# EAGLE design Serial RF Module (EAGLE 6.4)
DESCRIPTION: microOBD 200 OBD-II Module; HW_REV: 1.4; PCB_REV: C; PCB_SPEC1: Layer Count: 4; PCB_SPEC2: Size: 1.3" x 0.59"; PCB_SPEC3: Finish Thickness: 0.049" - 0.052"; PCB_SPEC4: Copper Weight: 1oz; TITLE: STM1120

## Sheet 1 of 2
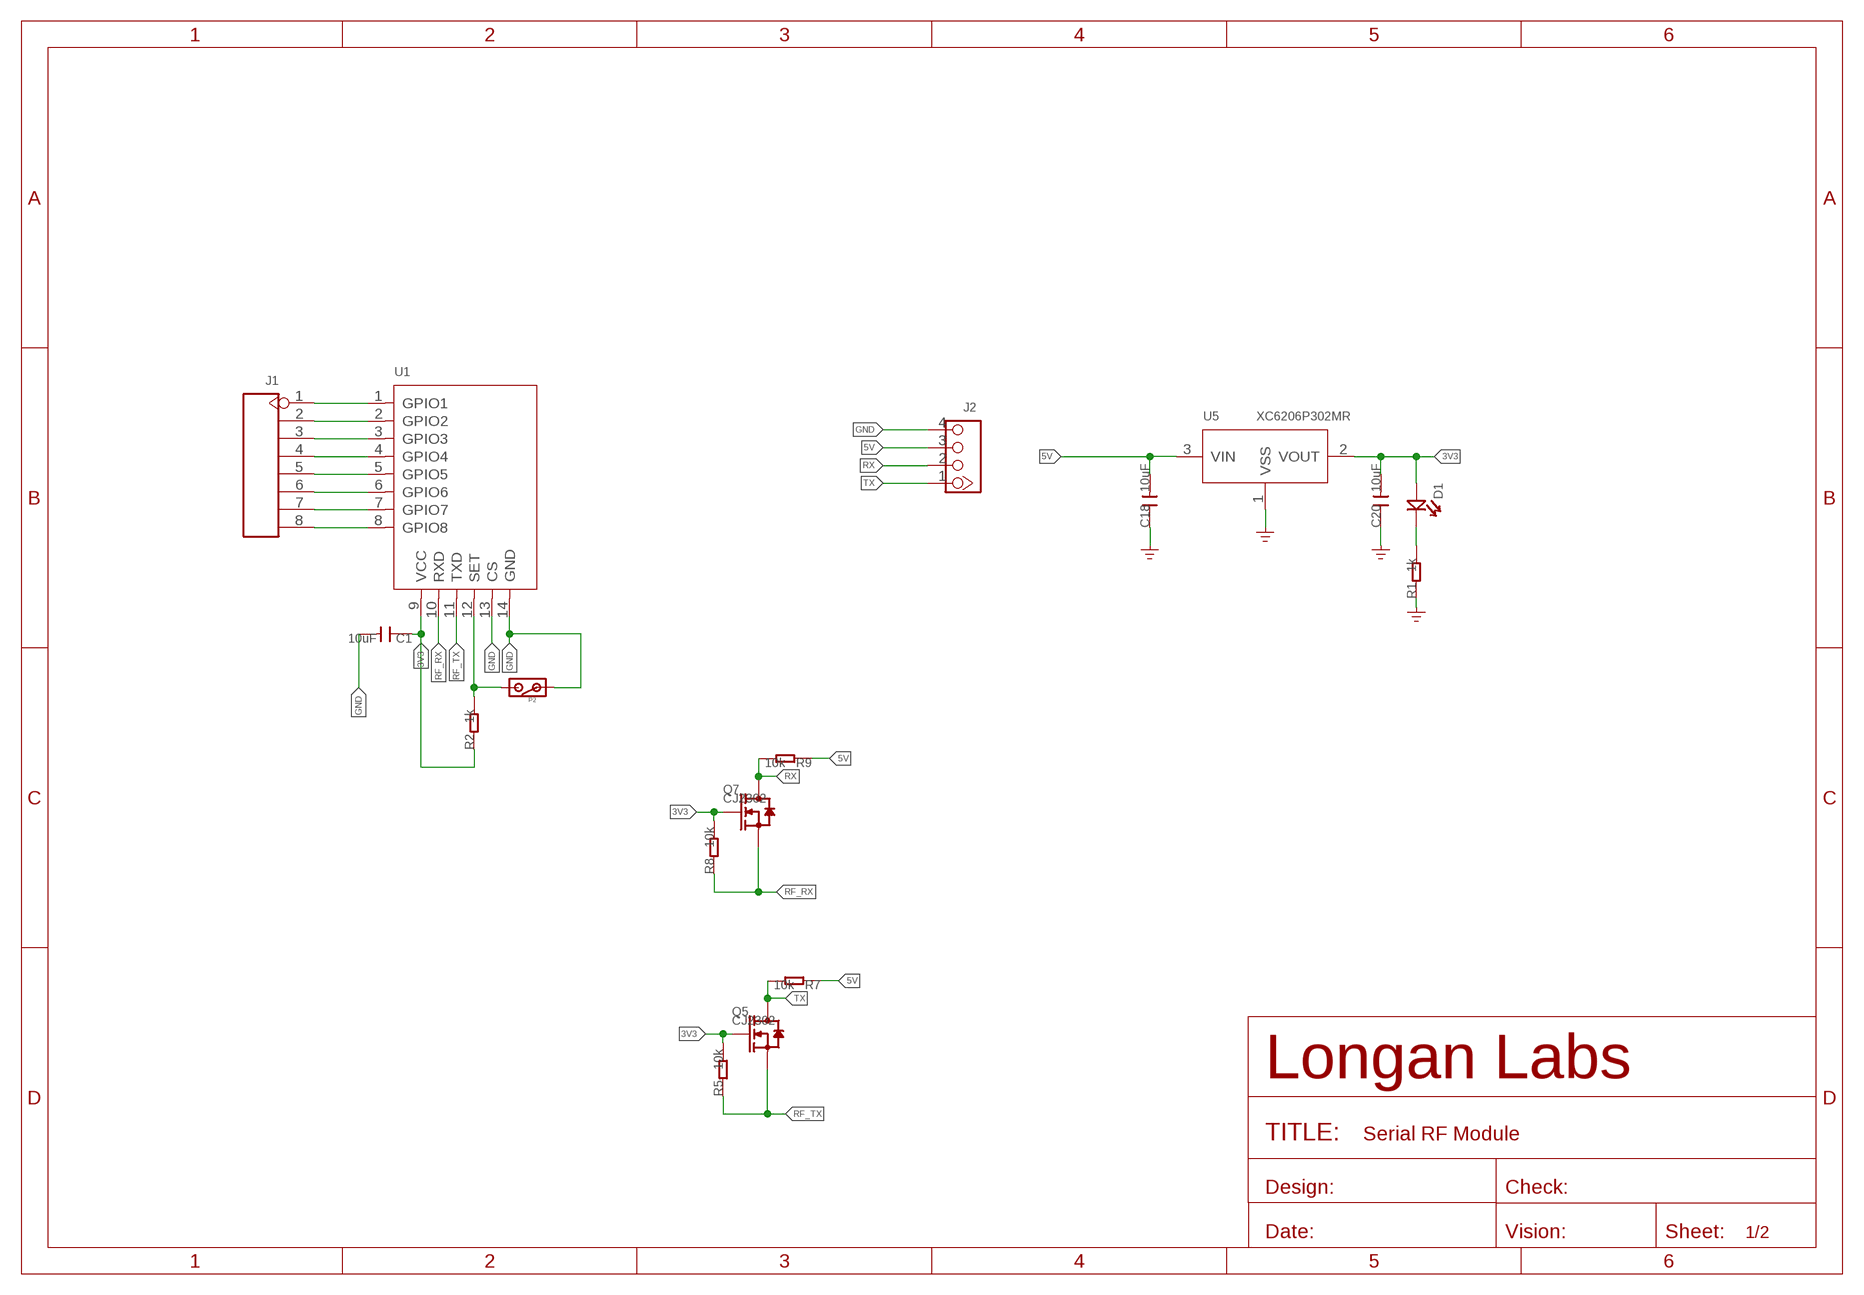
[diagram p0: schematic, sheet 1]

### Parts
C1  10uF  CAP-0603  [C0603]
C18  10uF  CAP-0603  [C0603]
C20  10uF  CAP-0603  [C0603]
D1  LED'0603'  [LED-0603]
J1  HEADER-8P-2.0-TEST  [H8-SMD-2.0-TEST]
J2  320110033  GROVE-CONNECTOR-DIP-2.0  [HW4-2.0]
P2  PAD-JUMPER-2P  [2P-SMD-1.78X1.27]
Q5  CJ2302  MOSFET-N'SOT23'  [SOT23]
Q7  CJ2302  MOSFET-N'SOT23'  [SOT23]
R1  1k  R-0603  [R0603]
R2  1k  R-0603  [R0603]
R5  10k  R-0603  [R0603]
R7  10k  R-0603  [R0603]
R8  10k  R-0603  [R0603]
R9  10k  R-0603  [R0603]
U1  MOUDLE-WIRELESS-SERIAL-JDY-40  [MOUDLE14P-1.5-23X13.7MM]
U5  XC6206P302MR  PMIC-XC6206PMR  [SOT-23]

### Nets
3V3: C1.1 C20.2 D1.+ Q5.1(G) Q7.1(G) R2.1 R5.2 R8.2 U1.9(VCC) U5.2(VOUT)
5V: C18.2 J2.3 R7.1 R9.1 U5.3(VIN)
GND: C1.2 C18.1 C20.1 J2.4 P2.1 R1.1 U1.13(CS) U1.14(GND) U5.1(VSS) ; supply symbol labelled GND_POWER
N$1: D1.- R1.2
N$2: P2.2 R2.2 U1.12(SET)
N$3: J1.1 U1.1(GPIO1)
N$4: J1.2 U1.2(GPIO2)
N$5: J1.3 U1.3(GPIO3)
N$6: J1.4 U1.4(GPIO4)
N$7: J1.5 U1.5(GPIO5)
N$8: J1.6 U1.6(GPIO6)
N$9: J1.7 U1.7(GPIO7)
N$10: J1.8 U1.8(GPIO8)
RF_RX: Q7.2(S) R8.1 U1.10(RXD)
RF_TX: Q5.2(S) R5.1 U1.11(TXD)
RX: J2.2 Q7.3(D) R9.2
TX: J2.1 Q5.3(D) R7.2

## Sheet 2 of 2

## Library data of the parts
C1 C18 C20 = Discrete-new:CAP: Ceramic Capacitors
D1 = Discrete-new:LED
J1 = Connector-new:HEADER-8P
J2 = Connector-new:GROVE-CONNECTOR-DIP: 4P-2.0:320110033;4P-2.0-90D:320110034
P2 = Discrete:PAD-JUMPER-2P
Q5 Q7 = Discrete:MOSFET-N: IRLL014: http://www.vishay.com/docs/91319/sihll014.pdf
R1 R2 R5 R7-R9 = Discrete:R*
U1 = Longan-moudle:MOUDLE-WIRELESS-SERIAL-JDY-40
U5 = IC-new:PMIC-XC6206P: LOW ESR Cap.Compatible Positive Voltage Regulators

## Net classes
3 usbvcc: width 0.152 mm, drill 0.152 mm, clearance 0.152 mm

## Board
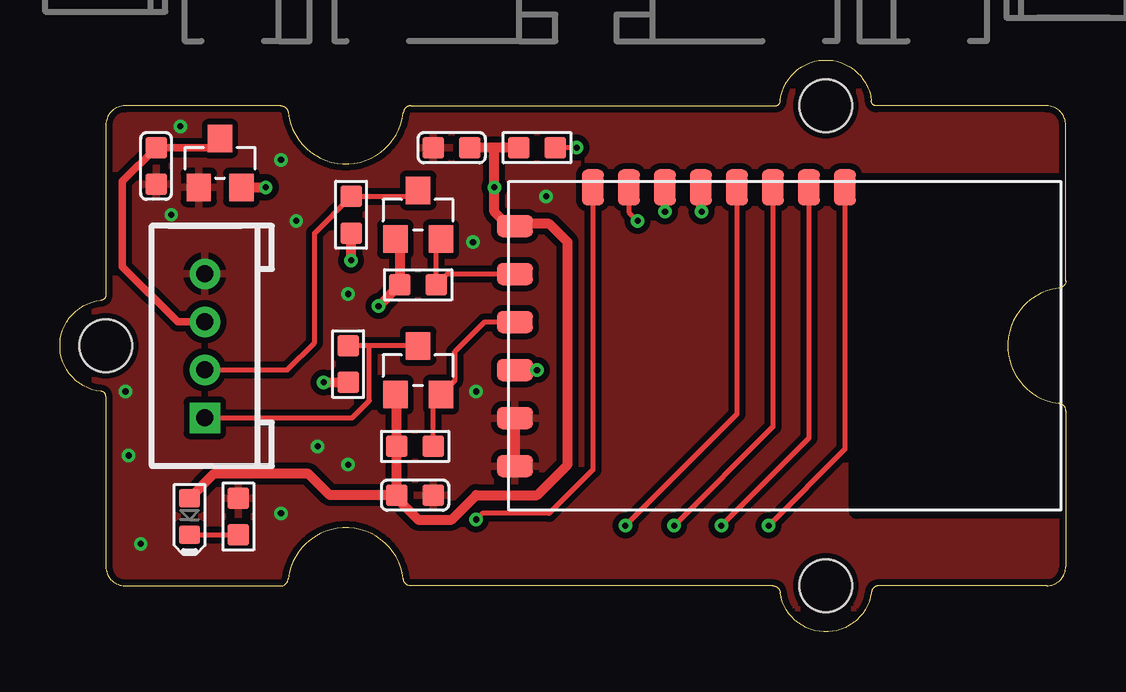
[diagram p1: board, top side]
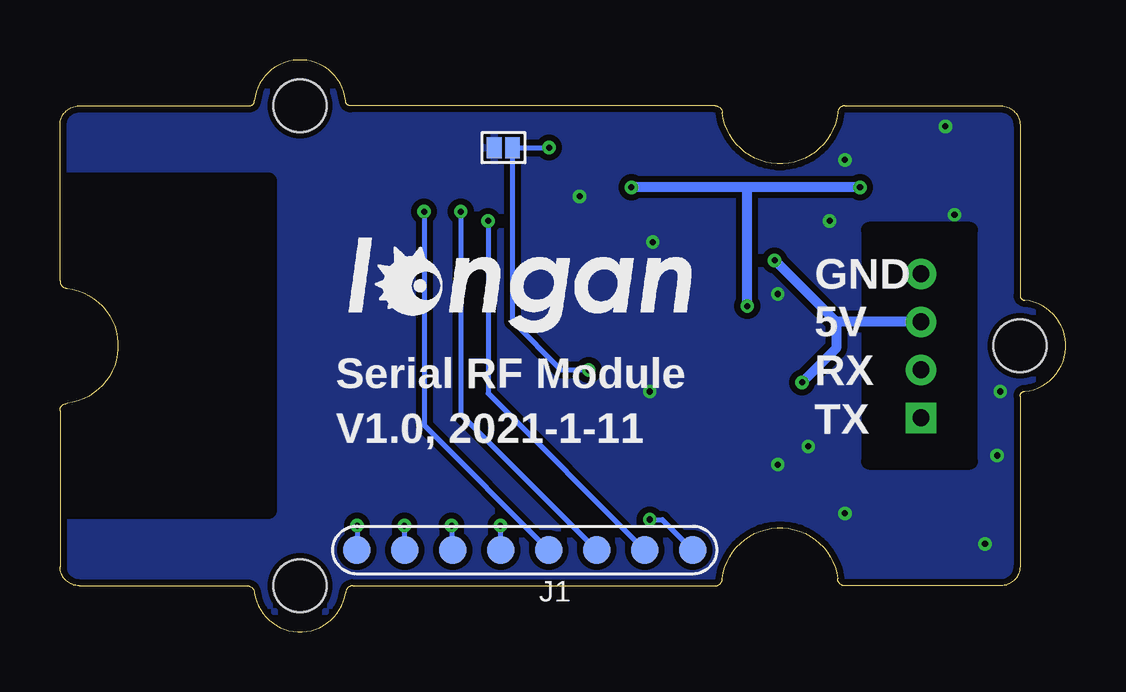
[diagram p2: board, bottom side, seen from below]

Size 41.91 x 23.83 mm. Coordinates in mm from the lower left corner, seen from the top.
Copper layers (1*16): Top 0.035mm / dielectric 1.5mm / Bottom 0.035mm
Design rules "SeeedStudio_2layer_DRU_no_angle_20140221 *": minimum track width 6mil, minimum drill 10mil, track to track 6mil, track to pad 6mil, pad to pad 6mil, via to via 6mil, smd to smd 0mil, copper to edge 10mil, drill to drill 10mil, minimum pad ring 10mil, minimum via ring 6mil, stop-mask expansion 2mil, vias tented up to drill 25mil, thermal gap 10mil
tRestrict: area 33.2,5.1 to 42.7,18.8
bRestrict: area 4,7.1 to 8.2,16.7; area 33.2,5.1 to 42.9,18.8

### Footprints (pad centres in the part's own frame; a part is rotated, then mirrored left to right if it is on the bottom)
C0603 = smd 0.889 x 0.889: 1 -0.762,0; 2 0.762,0
LED-0603 = smd 0.762 x 0.889: + 0.762,0; - -0.762,0
H8-SMD-2.0-TEST = smd 1.143 x 1.143: 1 0,7; 2 0,5; 3 0,3; 4 0,1; 5 0,-1; 6 0,-3; 7 0,-5; 8 0,-7
HW4-2.0 = drill 0.7 pad 1.27 square: 1 -3,0 | drill 0.7 pad 1.27: 2 -1,0; 3 1,0; 4 3,0
2P-SMD-1.78X1.27 = smd 0.889 x 0.61: 1 0,0.381; 2 0,-0.381
SOT23 = smd 1.016 x 1.143: 1 -0.95,-1.016; 2 0.95,-1.016; 3 0,1.016
R0603 = smd 0.889 x 0.889: 1 -0.762,0; 2 0.762,0
MOUDLE14P-1.5-23X13.7MM = smd 1.5 x 0.9: 1 -6.6,0; 2 -6.6,-1.5; 3 -6.6,-3; 4 -6.6,-4.5; 5 -6.6,-6; 6 -6.6,-7.5; 7 -6.6,-9; 8 -6.6,-10.5 | smd 0.9 x 1.5: 9 -4.985,-13.75; 10 -2.985,-13.75; 11 -0.985,-13.75; 12 1.015,-13.75; 13 3.015,-13.75; 14 5.015,-13.75
GROVE-TEST-PLATFORM = hole 2.2: -10,-10; -10,10; 20,0
SOT-23 = smd 1.016 x 1.143: 1 -0.889,-1.016; 2 0.889,-1.016; 3 0,1.016

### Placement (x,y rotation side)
C1  16.32,20.18 180 top
C18  4,19.41 90 top
C20  14.8,5.7 180 top
D1  5.4,4.81 90 top
J1  22.54,3.41 90 bottom
J2  6.03,11.92 90 top
P2  23.43,20.18 90 bottom
Q5  14.92,10.91 0 top
Q7  14.92,17.38 0 top
R1  7.43,4.81 270 top
R2  19.88,20.18 0 top
R5  14.8,7.73 180 top
R7  12,11.16 90 top
R8  14.92,14.46 180 top
R9  12.13,17.38 90 top
U1  32.7,11.92 270 top
U3  [GROVE-TEST-PLATFORM]  21.91,11.92 180 top
U5  6.67,19.54 0 top
U$5  [LONGAN-SILK-SMALLER]  31.18,11.29 0 bottom

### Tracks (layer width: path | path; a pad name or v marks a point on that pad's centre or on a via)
3V3  (via drill 0.25 pad 0.51)
  Top 0.406: U5.2 v8.57,18.53 | Q7.1 14.16,16.18 R8.2 v13.27,13.57 | C20.2 R5.2 14.03,9.83 Q5.1 | C20.2 11.24,5.7 10.35,6.59 6.41,6.59 D1.+ | R2.1 18.1,20.18 | 18.1,20.18 C1.1 | 18.1,20.18 v18.1,18.53 18.1,17.51 18.7,16.91 U1.9 19.05,17 20.38,17 21.15,16.24 21.15,6.97 19.88,5.7 17.34,5.7 16.32,4.68 14.92,4.68 14.03,5.57 C20.2
  Bottom 0.406: v8.57,18.53 13.27,18.53 | 13.27,18.53 v18.1,18.53 | v13.27,13.57 13.27,18.53
5V  (via drill 0.25 pad 0.51)
  Top 0.305: U5.3 6.29,20.18 C18.2 2.6,18.78 2.6,15.22 4.91,12.92 J2.3
  Top 0.406: v12.13,15.48 R9.1 | v10.99,10.4 R7.1
  Bottom 0.406: J2.3 9.57,12.92 | 9.57,12.92 v12.13,15.48 | 9.57,12.92 9.57,11.81 v10.99,10.4
GND  (via drill 0.25 pad 0.51)
  Top 0.406: U1.13 U1.14
  other vias: 12,14.08 9.21,19.67 12,6.97 2.73,10.02 4.64,17.38 9.84,17.13 9.21,4.94 10.73,7.73 17.21,16.24 17.34,10.02 3.37,3.67 2.86,7.35 20.26,18.14 5.02,21.07
  pour Bottom (isolate 0.254): -0.32,-0.14 42.23,-0.14 42.23,23.99 -0.32,23.99
  pour Top (isolate 0.254): -0.32,-0.14 42.23,-0.14 42.23,23.99 -0.32,23.99
N$1
  Top 0.203: D1.- R1.2
N$2  (via drill 0.25 pad 0.51)
  Top 0.203: U1.12 v19.88,10.91 | v21.53,20.18 R2.2
  Bottom 0.203: v19.88,10.91 21.02,10.91 23.05,12.94 P2.2 v21.53,20.18
N$3  (via drill 0.25 pad 0.51)
  Top 0.203: U1.1 32.7,7.6 v29.53,4.43
  Bottom 0.203: v29.53,4.43 29.53,3.43 J1.1
N$4  (via drill 0.25 pad 0.51)
  Top 0.203: U1.2 31.2,8.07 v27.56,4.43
  Bottom 0.203: v27.56,4.43 27.56,3.43 J1.2
N$5  (via drill 0.25 pad 0.51)
  Top 0.203: U1.3 29.7,8.54 v25.59,4.43
  Bottom 0.203: v25.59,4.43 25.59,3.46 J1.3
N$6  (via drill 0.25 pad 0.51)
  Top 0.203: U1.4 28.2,9.07 v23.56,4.43
  Bottom 0.203: v23.56,4.43 23.56,3.43 J1.4
N$7  (via drill 0.25 pad 0.51)
  Top 0.406: U1.5 26.7,17.54 v26.73,17.51
  Bottom 0.203: v26.73,17.51 26.73,8.6 J1.5
N$8  (via drill 0.25 pad 0.51)
  Top 0.203: U1.6 v25.2,17.52 v25.21,17.51
  Bottom 0.203: v25.21,17.51 25.21,9.08 J1.6
N$9  (via drill 0.25 pad 0.51)
  Top 0.203: U1.7 23.7,17.49 v24.07,17.13
  Bottom 0.203: v24.07,17.13 24.07,9.94 J1.7
N$10  (via drill 0.25 pad 0.51)
  Top 0.203: U1.8 22.2,6.76 20.38,4.94 17.59,4.94 v17.34,4.68
  Bottom 0.203: v17.34,4.68 16.81,4.68 J1.8
RF_RX
  Top 0.203: U1.10 16.13,14.91 R8.1 15.69,16.18 Q7.2
RF_TX
  Top 0.203: U1.11 17.69,12.91 16.45,11.67 16.45,10.46 Q5.2 15.56,9.57 R5.1
RX
  Top 0.203: J2.2 9.48,10.92 10.61,12.05 10.61,16.62 R9.2 14.67,18.14 Q7.3
TX
  Top 0.203: Q5.3 12.89,11.92 | 12.89,11.92 R7.2 | J2.1 12.18,8.92 12.89,9.64 12.89,11.92

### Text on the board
bPlace: GND | 5V | RX | Serial RF Module | TX | V1.0, 2021-1-11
